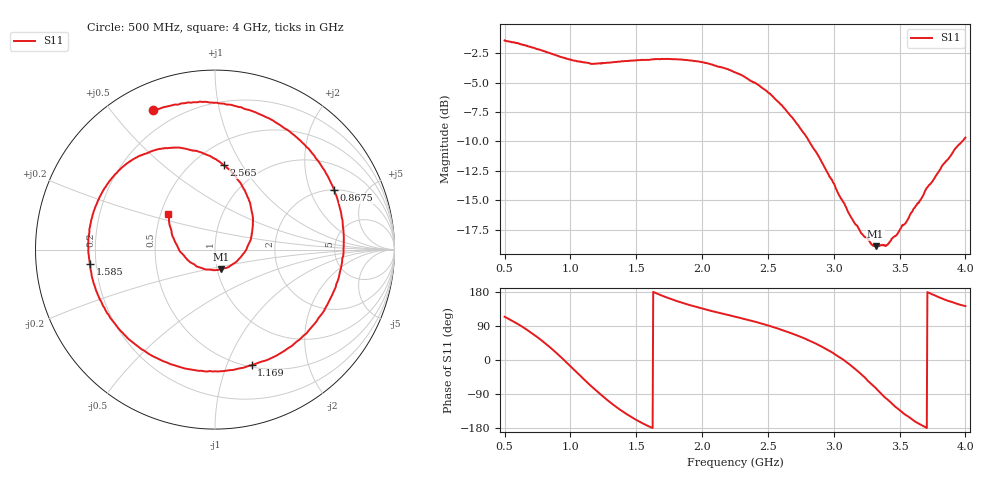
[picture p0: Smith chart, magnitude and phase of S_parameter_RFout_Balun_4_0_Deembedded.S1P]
!Agilent Technologies,E5071B,MY42403504,A.06.51
!Date: Wed Feb 26 14:55:32 2014
!Data & Calibration Information:
!Freq	S11:SOLT1(ON)
# Hz S dB R 50
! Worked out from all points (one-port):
!   801 points, 500 MHz to 4 GHz, reference 50 ohm
!   lowest |S11| = -18.9 dB at 3.317 GHz (marker M1), VSWR 1.26, Z = 52.1 - j11.5 ohm
!   |S11| at or under -10 dB: 2.814 GHz to 3.975 GHz (1.162 GHz wide, 34.2 % of centre)
!   S11 on the Smith chart (normalised r, x): 500 MHz: 0.12, +0.64; 867.5 MHz: 2.00, +2.97; 1.169 GHz: 0.52, -1.23; 1.585 GHz: 0.18, -0.06; 2.565 GHz: 0.69, +0.84; 4 GHz: 0.55, +0.25
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5e8  -1.42 114.0
6.00625e8  -1.66 94.9
6.925e8  -1.96 74.4
7.8e8  -2.26 52.0
8.675e8  -2.59 26.6
9.375e8  -2.85 4.5
9.9e8  -3.01 -13.0
1.0425e9  -3.15 -30.6
1.108125e9  -3.29 -52.9
1.169375e9  -3.41 -72.5
1.265625e9  -3.34 -101.5
1.375e9  -3.22 -130.6
1.475625e9  -3.12 -153.2
1.585e9  -3.07 -173.4
1.685625e9  -2.99 171.3
1.8125e9  -3.03 155.0
2.0225e9  -3.34 133.8
2.25e9  -4.13 114.3
2.420625e9  -5.15 99.4
2.565e9  -6.50 84.1
2.6875e9  -7.99 69.3
2.893125e9  -11.41 38.1
3.125e9  -16.31 -13.1
3.3175e9  -18.89 -73.4
3.409375e9  -18.76 -104.5
3.5625e9  -16.63 -148.5
3.811875e9  -12.32 163.9
4e9  -9.67 142.3
